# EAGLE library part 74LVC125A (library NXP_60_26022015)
Quad buffer/line driver with 5 V tolerant input/outputs; 3-state The 74LVC125A consists of four non-inverting buffers/line drivers with 3-state outputs (nY) that are controlled by the output enable input (nOE). A HIGH at nOE causes the outputs to assume a high-impedance OFF-state. Inputs can be driven from either 3.3 V or 5 V devices. When disabled, up to 5.5 V can be applied to the outputs. AAL Eindhoven MK
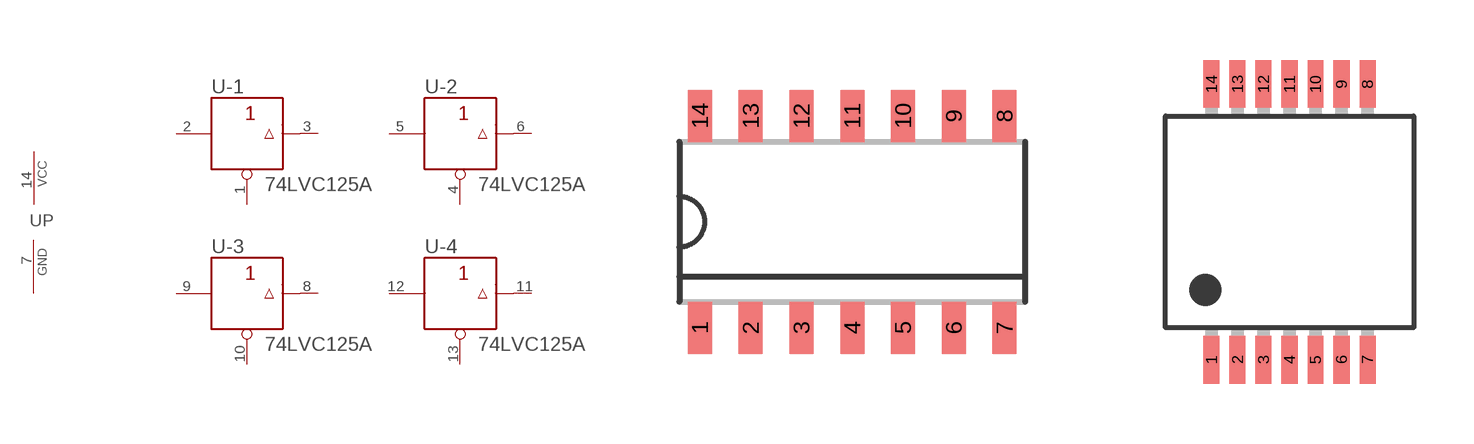
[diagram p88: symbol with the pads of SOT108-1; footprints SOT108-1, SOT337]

Designator prefix U; gates P=PWRN-1 -1=BUFFER_OE -2=BUFFER_OE -3=BUFFER_OE -4=BUFFER_OE

## 74LVC125AD (12NC: 9352 317 00118)  [SOT108-1]
1  -1:!OE  in
2  -1:A  in
3  -1:Y  out
4  -2:!OE  in
5  -2:A  in
6  -2:Y  out
7  P:GND  pwr
8  -3:Y  out
9  -3:A  in
10  -3:!OE  in
11  -4:Y  out
12  -4:A  in
13  -4:!OE  in
14  P:VCC  pwr

## 74LVC125ADB  [SOT337]
Pads as for SOT108-1

## 74LVC125APW  [SOT402-1]
Pads as for SOT108-1

## 74LVC125ABQ  [SOT762-1]
1  -1:!OE  in
2  -1:A  in
3  -1:Y  out
4  -2:!OE  in
5  -2:A  in
6  -2:Y  out
7  P:GND  pwr
8  -3:Y  out
9  -3:A  in
10  -3:!OE  in
11  -4:Y  out
12  -4:A  in
13  -4:!OE  in
14  P:VCC  pwr
CP  P:GND  pwr

## Footprint SOT108-1 (pad centres in mm)
SOT108-1 SO14: plastic small outline package; 14 leads; body width 3.9 mm; body thickness 1.47 mm JEDEC: MS-012 IEC: --
smd 0.6 x 1.3: 1 -3.81,-2.65; 2 -2.54,-2.65; 3 -1.27,-2.65; 4 0,-2.65; 5 1.27,-2.65; 6 2.54,-2.65; 7 3.81,-2.65; 8 3.81,2.65; 9 2.54,2.65; 10 1.27,2.65; 11 0,2.65; 12 -1.27,2.65; 13 -2.54,2.65; 14 -3.81,2.65

## Footprint SOT337 (pad centres in mm)
SOT337 SSOP14: plastic shrink small outline package; 14 leads; body width 5.3 mm JEDEC: MO-150 IEC: --
smd 0.4 x 1.2: 1 -1.95,-3.45; 2 -1.3,-3.45; 3 -0.65,-3.45; 4 0,-3.45; 5 0.65,-3.45; 6 1.3,-3.45; 7 1.95,-3.45; 8 1.95,3.45; 9 1.3,3.45; 10 0.65,3.45; 11 0,3.45; 12 -0.65,3.45; 13 -1.3,3.45; 14 -1.95,3.45

## Footprint SOT402-1 (pad centres in mm)
SOT402-1 TSSOP14: plastic thin shrink small outline package; 14 leads; body width 4.4 mm JEDEC: MO-153 IEC: ---
smd 0.6 x 1.35: 1 -2.05,-2.925; 7 2.05,-2.925; 8 2.05,2.925; 14 -2.05,2.925
smd 0.4 x 1.35: 2 -1.3,-2.925; 3 -0.65,-2.925; 4 0,-2.925; 5 0.65,-2.925; 6 1.3,-2.925; 9 1.3,2.925; 10 0.65,2.925; 11 0,2.925; 12 -0.65,2.925; 13 -1.3,2.925

## Footprint SOT762-1 (pad centres in mm)
SOT762-1 DHVQFN14: plastic dual in-line compatible thermal enhanced very thin quad flat package; no leads; 14 terminals; body 2.5 x 3 x 0.85 mm JEDEC: MO-241 IEC: -- JEITA: --
smd 1 x 0.29: 1 -1.5,-0.25; 7 1.5,-0.25; 8 1.5,0.25; 14 -1.5,0.25
smd 0.29 x 1: 2 -1,-1.35; 3 -0.5,-1.35; 4 0,-1.35; 5 0.5,-1.35; 6 1,-1.35; 9 1,1.35; 10 0.5,1.35; 11 0,1.35; 12 -0.5,1.35; 13 -1,1.35
smd 1.4 x 0.9: CP 0,0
